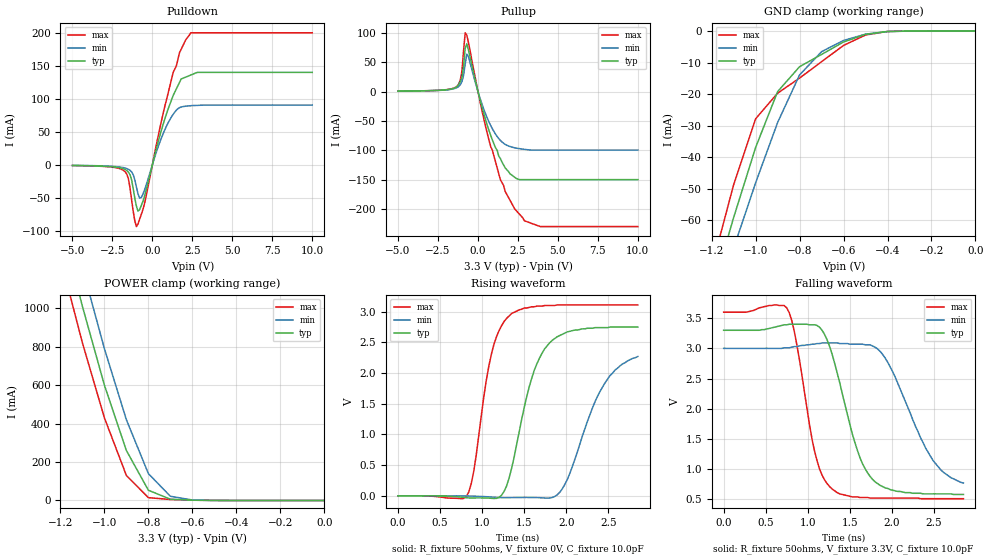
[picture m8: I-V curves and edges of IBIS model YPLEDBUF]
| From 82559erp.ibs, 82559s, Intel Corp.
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[Model]   YPLEDBUF
Model_type   I/O
Vinl  =   0.8V
Vinh  =   2.0V
|   typ   min   max
C_comp   3.0pF  NA   NA
| note : on die power/gnd supply distribution R/L/C
|   are not included in the simulation
| note : pull up and pull down mos are not active
|   pup#="1" pdn="0"
|variable   typ   min   max
[Voltage range]   3.3V   3.0V   3.6V
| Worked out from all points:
|   slope of the pulldown table from 0 to 0.495 V, typ, clamps not added: 10.7 ohm
|   slope of the pullup table from 0 to 0.495 V, typ, clamps not added: 9.93 ohm
|   GND clamp passes 1 mA (typ) near -0.49 V on its own axis
|   POWER clamp passes 1 mA (typ) near -0.56 V on its own axis
|   rising waveform, R_fixture 50ohms, V_fixture 0V, C_fixture 10.0pF: 20-80 % time 300ps typ, 384ps min, 220ps max; typ from 0 V to 2.75 V
|   falling waveform, R_fixture 50ohms, V_fixture 3.3V, C_fixture 10.0pF: 20-80 % time 321ps typ, 429ps min, 233ps max; typ from 3.3 V to 0.58 V
| note : all DC curves are with 0.2 OHM res. in series to the PAD.
[GND_clamp]
|Voltage   I(typ)   I(min)   I(max)
-5V       -1.11A     -990mA     -1.26A
-1.2V     -83.1mA    -90.4mA    -75mA
-1.1V     -59.1mA    -68.8mA    -48.7mA
-1V       -36.9mA    -48.1mA    -27.8mA
-900mV    -19.2mA    -29mA      -19.7mA
-800mV    -11.3mA    -13.9mA    -14.9mA
-700mV    -7.42mA    -6.54mA    -9.72mA
-600mV    -3.47mA    -2.98mA    -4.56mA
-500mV    -1.05mA    -990uA     -1.27mA
-400mV    -150uA     -180uA     -130uA
0V        0A         0A         0A
[PullDown]
| Voltage   I(typ)   I(min)   I(max)
-5V       -1.09mA    -920uA     -1.22mA
-1.7V     -7.22mA    -5mA       -10.7mA
-1.5V     -11.1mA    -6.86mA    -21mA
-1.3V     -22.7mA    -10.8mA    -53mA
-1V       -62.5mA    -33.6mA    -93.7mA
-800mV    -68.2mA    -50.6mA    -82.6mA
-600mV    -56.1mA    -45.1mA    -68.7mA
500mV     46.9mA     36.4mA     59mA
1.3V      105mA      76.5mA     140mA
1.8V      130mA      87.5mA     175mA
2.4V      136mA      89.5mA     200mA
10V       140mA      90.5mA     200mA
[POWER_clamp]
| Voltage   I(typ)   I(min)   I(max)
-5V       20.1A      20.2A      19.9A
-1.2V     1.45A      1.65A      1.26A
-1.1V     1.01A      1.21A      820mA
-1V       600mA      790mA      430mA
-900mV    260mA      420mA      130mA
-800mV    53.3mA     140mA      14.7mA
-700mV    6.62mA     21.9mA     5.15mA
-600mV    1.55mA     2.51mA     1.53mA
0V        1.7uA      1.91uA     1.49uA
[PullUp]
| Voltage   I(typ)   I(min)   I(max)
-5V       770uA      740uA      780uA
-1.3V     8.91mA     6.9mA      9.37mA
-1V       24.4mA     17.3mA     35.6mA
-800mV    73.6mA     46.6mA     100mA
-700mV    81.2mA     63.7mA     96.1mA
-600mV    71.3mA     59.6mA     84mA
400mV     -41.1mA    -32.8mA    -50.6mA
1.4V      -114mA     -83.2mA    -150mA
2V        -140mA     -93.6mA    -185mA
2.9V      -150mA     -98.5mA    -220mA
3.9V      -150mA     -99.8mA    -230mA
10V       -150mA     -99.8mA    -230mA
[Ramp]
| note : pad parasitics are not included
|Variable   typ   min   max
dV/dt_r   1.66/0.15n   1.42/0.21n   1.63/0.10n
dV/dt_f   1.63/0.16n   1.40/0.25n   1.85/0.12n
R_load =   50ohms
[Rising Waveform]
| note : pad parasitics are not included
| note : input changes at T=0.03nS
R_fixture   = 50ohms
V_fixture   = 0V
C_fixture   = 10.0pF
|Time   typ(V)   min(V)   max(V)
0s        4.71nV     4.32nV     2.7nV
810ps     -30.7mV    -2.55mV    -14.99mV
900ps     -34.5mV    -5.72mV    400mV
1.11ns    -40.6mV    -19.65mV   2.31V
1.35ns    450mV      -29.45mV   2.97V
1.59ns    1.92V      -27.45mV   3.08V
1.8ns     2.49V      -36.42mV   3.1V
2.01ns    2.67V      260mV      3.11V
2.46ns    2.74V      1.84V      3.11V
2.85ns    2.75V      2.27V      3.11V
[Falling Waveform]
| note : pad parasitics are not included
| note : input changes at T=0.03nS
R_fixture   = 50ohms
V_fixture   = 3.3V
V_fixture_min   = 3.0V
V_fixture_max   = 3.6V
C_fixture   = 10.0pF
|Time   typ   min   max
0s        3.3V       3V         3.6V
750ps     3.39V      3.01V      3.67V
840ps     3.4V       3.03V      3.28V
1.08ns    3.39V      3.07V      1.3V
1.29ns    2.9V       3.09V      670mV
1.59ns    1.31V      3.07V      540mV
1.77ns    830mV      3.04V      520mV
1.95ns    680mV      2.77V      520mV
2.49ns    590mV      1.14V      510mV
2.85ns    580mV      770mV      510mV
